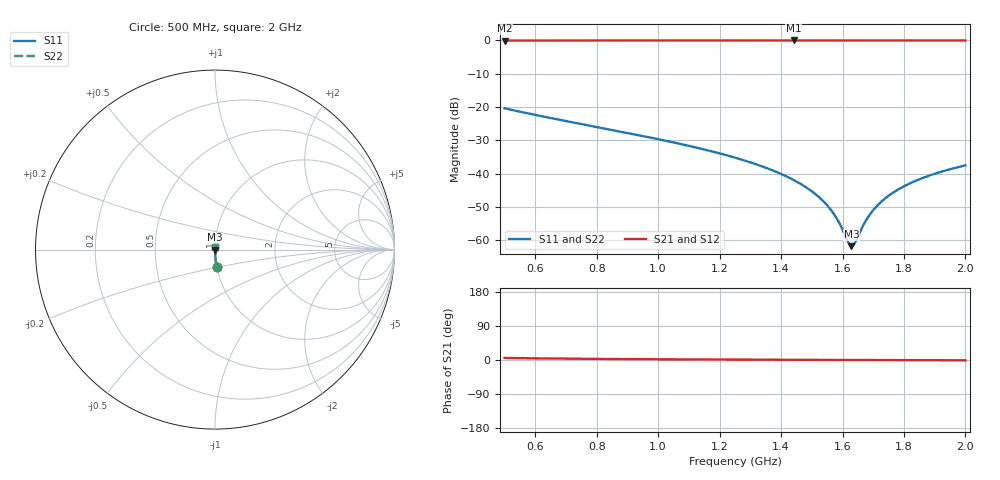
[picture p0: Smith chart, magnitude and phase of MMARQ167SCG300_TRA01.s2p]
! MMARQ167SCG300_TRA01  S-PARAMETER MODEL  ( General Type )
! Model Generated by TAIYO YUDEN Corporation (http://www.ty-top.com)
! Version 1.0
! TAIYO YUDEN Control No. 160201
! Copyright(c) 2016 TAIYO YUDEN CO.,LTD. All Rights Reserved.
! Product Description (link to TY-COMPAS)
! https://ds.yuden.co.jp/TYCOMPAS/or/detail?pn=MMARQ167SCG300JTRA01&u=M
! Products Name : Multilayer Ceramic Capacitors
! Characteristics :
!  Capacitance : 30 pF , Rated Voltage : 250V , TCC : CG / C0G
!  Case Size : 1.6 x 0.8 / 0.063 x 0.031 [mm/inch] , Thickness : 0.7 / 0.028 [mm/inch]
!  (Conditions: Temperature = 25 degC , DC Bias Current/Voltage = 0A / 0V)
! External Node Assignments :
!  1  o---| |---o  2
! GND o---------o GND
! Frequency Range : 500MHz  -  2000MHz  [ 401 STEP ]
# MHz S RI R 50
! Freq[MHz].  S11 Real  S11 Imag  S21 Real  S21 Imag  S12 Real  S12 Imag  S22 Real  S22 Imag
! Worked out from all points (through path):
!   401 points, 500 MHz to 2 GHz, reference 50 ohm
!   highest |S21| = -0.01 dB at 1.441 GHz (marker M1); lowest = 0.0 dB at 500 MHz (marker M2)
!   group delay of S21, straight-line fit = 10.1 ps
!   lowest |S11| = -61.8 dB at 1.629 GHz (marker M3), VSWR 1.00, Z = 50.1 - j0.00553 ohm
!   |S11| at or under -10 dB: start of sweep to end of sweep
!   |S22| runs from -61.8 to -20.4 dB; largest |S21 - S12| = 0
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500  0.00952 -0.0952  0.9905 0.0952  0.9905 0.0952  0.00952 -0.0952
751.25  0.00354 -0.0553  0.9965 0.0553  0.9965 0.0553  0.00354 -0.0553
1002.5  0.00165 -0.0327  0.9984 0.0327  0.9984 0.0327  0.00165 -0.0327
1137.5  0.0012 -0.0238  0.9988 0.0238  0.9988 0.0238  0.0012 -0.0238
1250  0.00098 -0.0174  0.999 0.0174  0.999 0.0174  0.00098 -0.0174
1358.75  0.00086 -0.0118  0.9991 0.0118  0.9991 0.0118  0.00086 -0.0118
1441.25  0.000814 -0.00798  0.9992 0.00798  0.9992 0.00798  0.000814 -0.00798
1501.25  0.0008 -0.00533  0.9992 0.00533  0.9992 0.00533  0.0008 -0.00533
1535  0.000799 -0.00389  0.9992 0.00389  0.9992 0.00389  0.000799 -0.00389
1565  0.000801 -0.00264  0.9992 0.00264  0.9992 0.00264  0.000801 -0.00264
1587.5  0.000804 -0.00171  0.9992 0.00171  0.9992 0.00171  0.000804 -0.00171
1617.5  0.000812 -0.000503  0.9992 0.000503  0.9992 0.000503  0.000812 -0.000503
1628.75  0.000815 -5.53e-05  0.9992 5.53e-05  0.9992 5.53e-05  0.000815 -5.53e-05
1640  0.000819 0.000389  0.9992 -0.000389  0.9992 -0.000389  0.000819 0.000389
1670  0.000831 0.00156  0.9992 -0.00156  0.9992 -0.00156  0.000831 0.00156
1692.5  0.000841 0.00242  0.9992 -0.00242  0.9992 -0.00242  0.000841 0.00242
1718.75  0.000855 0.00342  0.9991 -0.00342  0.9991 -0.00342  0.000855 0.00342
1752.5  0.000876 0.00467  0.9991 -0.00467  0.9991 -0.00467  0.000876 0.00467
1797.5  0.000907 0.00631  0.9991 -0.00631  0.9991 -0.00631  0.000907 0.00631
1853.75  0.000952 0.00831  0.999 -0.00831  0.999 -0.00831  0.000952 0.00831
1925  0.00102 0.0108  0.999 -0.0108  0.999 -0.0108  0.00102 0.0108
2000  0.0011 0.0133  0.9989 -0.0133  0.9989 -0.0133  0.0011 0.0133
